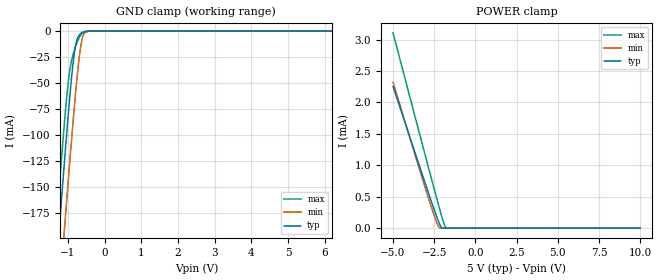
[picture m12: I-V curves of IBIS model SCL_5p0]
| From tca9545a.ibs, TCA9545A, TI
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|   Model
[Model]   SCL_5p0
Model_type   Input
Vinl = 1.5
Vinh = 3.5
|   typ   min   max
C_comp   3.453pF   3.557pF   3.722pF
[Voltage Range]   5   4.5   5.5
[Temperature Range]   27   125   -40
[Power Clamp Reference]   5   4.5   5.5
[GND Clamp Reference]   -0   -0   -0
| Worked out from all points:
|   GND clamp passes 1 mA (typ) near -0.59 V on its own axis
|   POWER clamp passes 1 mA (typ) near -3.41 V on its own axis
[GND Clamp]
|   Voltage   I(typ)   I(min)   I(max)
-5V       -2.043A    -2.104A    -2.005A
-1.43V    -283.8mA   -349.6mA   -242.9mA
-1.25V    -198.7mA   -264.5mA   -158.3mA
-1.235V   -191.7mA   -257.4mA   -151.5mA
-1.13V    -143.3mA   -208.6mA   -104.4mA
-1.085V   -123mA     -187.9mA   -85.34mA
-965mV    -71.2mA    -133.8mA   -42.55mA
-830mV    -23.15mA   -76.23mA   -19.53mA
-770mV    -10.86mA   -52.74mA   -13.07mA
-680mV    -3.519mA   -22.77mA   -5.653mA
-575mV    -759.6uA   -3.738mA   -1.166mA
9.985V    0A         0A         0A
[POWER Clamp]
|   Voltage   I(typ)   I(min)   I(max)
-5V       2.254mA    2.322mA    3.108mA
-3.155V   796.5uA    731.5uA    1.266mA
-2.435V   243.8uA    145.9uA    556.9uA
-2.255V   115.1uA    32.61uA    383uA
-2.18V    66.36uA    8.183uA    311.6uA
-2.09V    19.52uA    710nA      227.2uA
-1.91V    7.641nA    0A         69.73uA
-1.805V   0A         0A         7.88uA
9.985V    0A         0A         0A
